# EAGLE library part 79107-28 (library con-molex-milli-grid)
RECEPTACAL
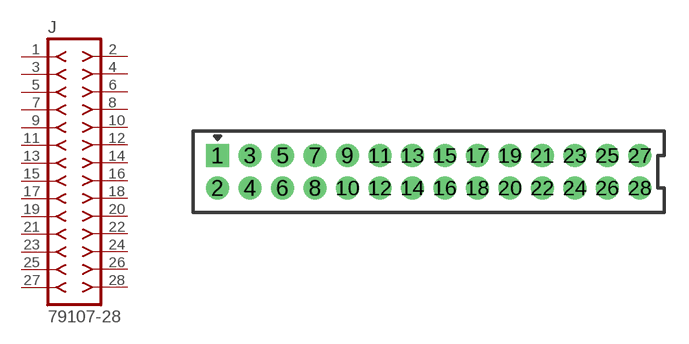
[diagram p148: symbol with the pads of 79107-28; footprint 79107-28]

Designator prefix J

## 79107-28  [79107-28]
1  1  pas
2  2  pas
3  3  pas
4  4  pas
5  5  pas
6  6  pas
7  7  pas
8  8  pas
9  9  pas
10  10  pas
11  11  pas
12  12  pas
13  13  pas
14  14  pas
15  15  pas
16  16  pas
17  17  pas
18  18  pas
19  19  pas
20  20  pas
21  21  pas
22  22  pas
23  23  pas
24  24  pas
25  25  pas
26  26  pas
27  27  pas
28  28  pas

## Footprint 79107-28 (pad centres in mm)
RECEPTACAL Dual Row, Vertical, Through-Hole
drill 0.914 square: 1 -13,1
drill 0.914: 2 -13,-1; 3 -11,1; 4 -11,-1; 5 -9,1; 6 -9,-1; 7 -7,1; 8 -7,-1; 9 -5,1; 10 -5,-1; 11 -3,1; 12 -3,-1; 13 -1,1; 14 -1,-1; 15 1,1; 16 1,-1; 17 3,1; 18 3,-1; 19 5,1; 20 5,-1; 21 7,1; 22 7,-1; 23 9,1; 24 9,-1; 25 11,1; 26 11,-1; 27 13,1; 28 13,-1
